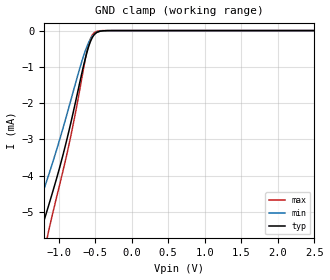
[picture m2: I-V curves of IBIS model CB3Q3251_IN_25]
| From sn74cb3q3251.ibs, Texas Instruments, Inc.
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[Model]   CB3Q3251_IN_25
Model_type  Input
Vinl=0.7
Vinh=1.7
| variable   typ   min   max
C_comp   2.62pF   2.35pF   2.78pF
[Temperature Range]   40   100   -40
| Ambient temperature   25   85   -40
[Voltage range]   2.5   2.3   2.7
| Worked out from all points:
|   GND clamp passes 1 mA (typ) near -0.66 V on its own axis
[GND Clamp]
| CB3Q3251_IN_25
|   Voltage   I(typ)   I(min)   I(max)
-5.5V     -49.44mA   -39.07mA   -64.15mA
-1.395V   -6.705mA   -5.604mA   -8.313mA
-1.245V   -5.549mA   -4.642mA   -6.598mA
-1.14V    -4.845mA   -4.006mA   -5.56mA
-985mV    -3.768mA   -3mA       -4.242mA
-865mV    -2.819mA   -2.154mA   -3.207mA
-710mV    -1.426mA   -1.035mA   -1.622mA
-615mV    -618uA     -451.2uA   -591.9uA
-565mV    -305.7uA   -235.1uA   -229.6uA
-515mV    -119uA     -101.9uA   -63.96uA
-335mV    -1.066uA   -1.71uA    -103.1nA
2.5V      55pA       199pA      20.15pA
